(* Logix 5000 DataType export AMCI_Motion_Axis_Output_Data; software revision 20.03 *)

TYPE AMCI_Motion_Axis_Output_Data :
STRUCT
   Control_Word_0 : INT;
   Control_Word_1 : INT;
   Position_or_Distance : DINT;
   Programmed_Speed : DINT;
   Acceleration : INT;
   Deceleration : INT;
   Output_Word_8 : INT;
   Output_Word_9 : INT;
END_STRUCT
END_TYPE
